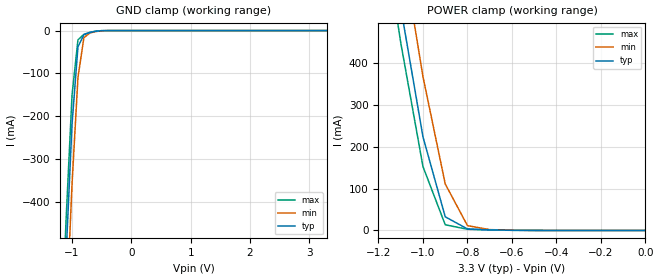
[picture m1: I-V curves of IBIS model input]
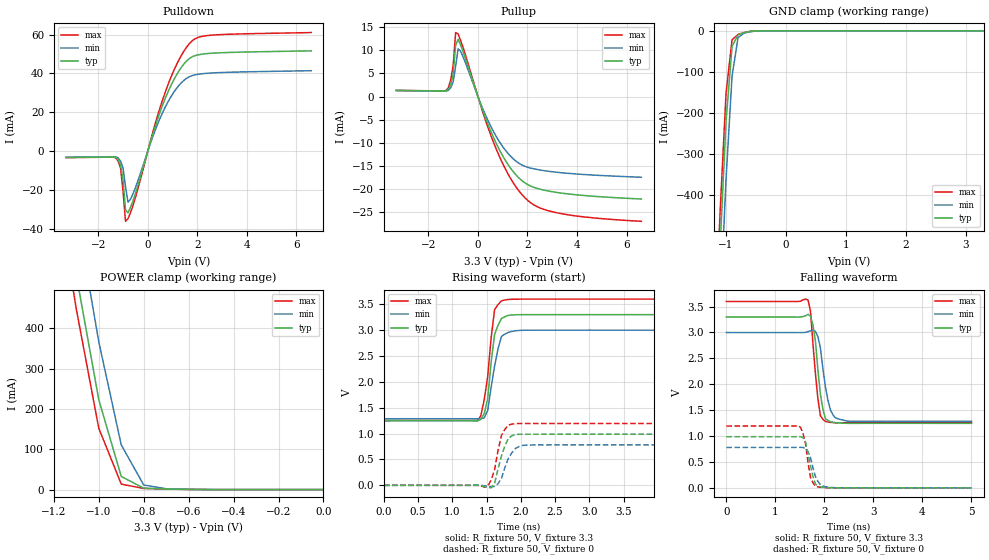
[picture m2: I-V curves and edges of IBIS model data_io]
| TSOP package &  Commercial  Operation
[IBIS Ver]   3.2
[Comment Char]   |_char
[File name]   as7c31026b_tsopc.ibs
[File Rev]   1.0
[Date]   May 19, 2004 3:47:46 PM
[Source]
Alliance Semiconductor Corporation
[Notes]
This model  is for TSOP package &
 Commercial  Operation
[Disclaimer]
Data is for modeling purpose only and is not guaranted.
This IBIS model is provided on an "AS IS" basis and Alliance Semiconductor makes
absolutely no warranty with respect to the information contained
herein.The entire risk as to quality and performance
is with the Customer. ACCORDINGLY, IN NO EVENT SHALL THE COMPANY BE
LIABLE FOR ANY DAMAGES, WHETHER IN CONTRACT OR TORT,INCLUDING ANY
LOST PROFITS OR OTHER INCIDENTAL, CONSEQUENTIAL, EXEMPLARY, OR
PUNITIVE DAMAGES ARISING OUT OF THE USE OR APPLICATION OF THE IBIS
model provided in this package.
[Copyright]
Alliance Semiconductor Corporation
| TSOP Package & Commercial Operation.
[Component]   AS7C31026B_TSOPC
Si_location Pin
Timing_location Pin
[Manufacturer]   Alliance Semiconductor Corporation
[Package]
R_pkg   321.15m   142.5m   499.8m
L_pkg   5.882nH   2.534nH   9.23nH
C_pkg   1.013pF   0.614pF   1.412pF
[Pin] signal_name   model_name
1   A4   input
2   A3   input
3   A2   input
4   A1   input
5   A0   input
6   NCE   input
7   IO0   data_io
8   IO1   data_io
9   IO2   data_io
10   IO3   data_io
11   VCC   POWER
12   GND   GND
13   IO4   data_io
14   IO5   data_io
15   IO6   data_io
16   IO7   data_io
17   NWE   input
18   A15   input
19   A14   input
20   A13   input
21   A12   input
22   NC   NC
23   NC   NC
24   A11   input
25   A10   input
26   A9   input
27   A8   input
28   NC   NC
29   IO8   data_io
30   IO9   data_io
31   IO10   data_io
32   IO11   data_io
33   VCC   POWER
34   GND   GND
35   IO12   data_io
36   IO13   data_io
37   IO14   data_io
38   IO15   data_io
39   NLB   input
40   NUB   input
41   NOE   input
42   A7   input
43   A6   input
44   A5   input
| Models and submodels in the file (2): input (Input), data_io (I/O)
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[Model]   input
Model_type Input
Vinh=2V
Vinl=0.8V
C_comp   4pF   4pF   4pF
[Model Spec]
[Temperature Range] 25   70   0
[Voltage Range]   3.3   3.0   3.6
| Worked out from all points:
|   GND clamp passes 1 mA (typ) near -0.56 V on its own axis
|   POWER clamp passes 1 mA (typ) near -0.65 V on its own axis
[GND Clamp]
-3.3V     -8.605A    -8.678A    -8.569A
-1.2V     -871.8mA   -1.032A    -786.6mA
-1.1V     -525.3mA   -681.9mA   -442.6mA
-1V       -219.6mA   -359.8mA   -151.4mA
-900mV    -38.16mA   -110mA     -21.74mA
-800mV    -9.652mA   -16.68mA   -8.786mA
-700mV    -4.621mA   -5.631mA   -4.129mA
-600mV    -1.581mA   -2.258mA   -1.211mA
-400mV    -22.59uA   -71.08uA   -10.05uA
3.3V      156pA      1.566uA    81.03pA
[POWER Clamp]
-3.3V     8.613A     8.687A     8.576A
-1.2V     879.9mA    1.042A     793.6mA
-1.1V     531.7mA    690.5mA    447.6mA
-1V       222.9mA    366.4mA    152.1mA
-900mV    32.63mA    110.9mA    13.56mA
-800mV    3.618mA    11.48mA    2.851mA
-700mV    1.463mA    2.037mA    1.288mA
0V        156pA      1.542nA    96.3pA
[Model]   data_io
Model_type I/O
Enable Active-High
Polarity Non-Inverting
Vinh=2V
Vinl=0.8V
Vref=1.728V
Vmeas=1.5V
Rref=168
Cref=30pF
C_comp   4pF   4pF   4pF
[Temperature Range] 25   70   0
[Voltage Range]   3.3   3.0   3.6
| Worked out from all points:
|   slope of the pulldown table from 0 to 0.495 V, typ, clamps not added: 24.6 ohm
|   slope of the pullup table from 0 to 0.495 V, typ, clamps not added: 68.8 ohm
|   GND clamp passes 1 mA (typ) near -0.56 V on its own axis
|   POWER clamp passes 1 mA (typ) near -0.65 V on its own axis
|   falling waveform, R_fixture 50, V_fixture 3.3: 20-80 % time 137ps typ, 165ps min, 129ps max; typ from 3.3 V to 1.25 V
|   falling waveform, R_fixture 50, V_fixture 0: 20-80 % time 138ps typ, 152ps min, 120ps max; typ from 0.987 V to 0.001 V
|   rising waveform, R_fixture 50, V_fixture 3.3: 20-80 % time 101ps typ, 134ps min, 119ps max; typ from 1.25 V to 3.3 V
|   rising waveform, R_fixture 50, V_fixture 0: 20-80 % time 131ps typ, 144ps min, 115ps max; typ from 0 V to 0.988 V
[Pullup]
-3.3V     1.309mA    1.298mA    1.319mA
-1.3V     1.177mA    1.139mA    1.277mA
-1.1V     2.464mA    1.876mA    3.58mA
-1V       4.894mA    3.142mA    6.707mA
-900mV    11.13mA    6.531mA    13.83mA
-800mV    12.37mA    10.31mA    13.53mA
-700mV    11.15mA    9.779mA    12.14mA
700mV     -9.696mA   -8.272mA   -10.85mA
1.3V      -15.38mA   -12.82mA   -17.55mA
1.9V      -18.69mA   -15.11mA   -21.92mA
3.2V      -20.76mA   -16.4mA    -25.17mA
6.6V      -22.17mA   -17.47mA   -27mA
[Pulldown]
-3.3V     -3.25mA    -3.145mA   -3.291mA
-1.3V     -3.123mA   -2.838mA   -3.453mA
-1.1V     -7.003mA   -5.036mA   -8.672mA
-1V       -14.54mA   -8.664mA   -20.63mA
-900mV    -30.21mA   -18.24mA   -36.08mA
-800mV    -31.71mA   -26.22mA   -34.76mA
-700mV    -28.96mA   -24.78mA   -31.66mA
700mV     27.02mA    22.56mA    30.19mA
1.2V      40.13mA    32.95mA    45.56mA
1.7V      47.87mA    38.44mA    55.66mA
2.6V      50.42mA    40.25mA    59.72mA
6.6V      51.64mA    41.41mA    61.03mA
[GND Clamp]
-3.3V     -8.605A    -8.678A    -8.569A
-1.2V     -871.8mA   -1.032A    -786.6mA
-1.1V     -525.3mA   -681.9mA   -442.6mA
-1V       -219.6mA   -359.8mA   -151.4mA
-900mV    -38.16mA   -110mA     -21.74mA
-800mV    -9.652mA   -16.68mA   -8.786mA
-700mV    -4.621mA   -5.631mA   -4.129mA
-600mV    -1.581mA   -2.258mA   -1.211mA
-400mV    -22.59uA   -71.08uA   -10.05uA
3.3V      156pA      1.566uA    81.03pA
[POWER Clamp]
-3.3V     8.613A     8.687A     8.576A
-1.2V     879.9mA    1.042A     793.6mA
-1.1V     531.7mA    690.5mA    447.6mA
-1V       222.9mA    366.4mA    152.1mA
-900mV    32.63mA    110.9mA    13.56mA
-800mV    3.618mA    11.48mA    2.851mA
-700mV    1.463mA    2.037mA    1.288mA
0V        156pA      1.542nA    96.3pA
[Falling Waveform]
R_fixture=50
V_fixture=3.3
V_fixture_min=3.0
V_fixture_max=3.6
0s        3.3V       3V         3.6V
1.667ns   3.351V     3.017V     3.628V
1.717ns   3.312V     3.032V     3.402V
1.768ns   3.14V      3.048V     2.771V
1.869ns   2.263V     2.916V     1.713V
1.919ns   1.806V     2.699V     1.39V
2.02ns    1.339V     1.954V     1.283V
2.121ns   1.279V     1.51V      1.265V
2.323ns   1.253V     1.32V      1.256V
5ns       1.247V     1.288V     1.255V
[Falling Waveform]
R_fixture=50
V_fixture=0
V_fixture_min=0
V_fixture_max=0
0s        987.1mV    780.3mV    1.194V
1.465ns   991.4mV    782.8mV    1.199V
1.515ns   988.3mV    783.2mV    1.167V
1.616ns   884.2mV    759.7mV    851mV
1.667ns   650.4mV    697.8mV    480.1mV
1.717ns   425.3mV    587.2mV    200.8mV
1.818ns   72.24mV    218mV      30.49mV
1.919ns   18.85mV    61.55mV    11.86mV
2.172ns   3.007mV    6.68mV     1.845mV
5ns       1.203mV    1.221mV    1.233mV
[Rising Waveform]
R_fixture=50
V_fixture=3.3
V_fixture_min=3.0
V_fixture_max=3.6
0s        1.246V     1.287V     1.254V
1.364ns   1.244V     1.286V     1.253V
1.414ns   1.273V     1.289V     1.339V
1.465ns   1.383V     1.303V     1.653V
1.515ns   1.672V     1.446V     2.098V
1.566ns   2.377V     1.893V     2.85V
1.616ns   2.915V     2.304V     3.393V
1.717ns   3.224V     2.878V     3.564V
2.02ns    3.298V     2.996V     3.598V
5ns       3.298V     2.998V     3.598V
[Rising Waveform]
R_fixture=50
V_fixture=0
V_fixture_min=0
V_fixture_max=0
0s        0V         0V         0V
1.515ns   -39.5mV    -15.58mV   -16.28mV
1.566ns   -47.94mV   -27.89mV   101.8mV
1.616ns   36.55mV    -19.97mV   302mV
1.717ns   571.3mV    136.7mV    965.1mV
1.818ns   909.9mV    523.2mV    1.166V
1.869ns   956.2mV    630.6mV    1.183V
1.97ns    986.7mV    748.6mV    1.194V
2.121ns   987.9mV    779mV      1.194V
5ns       988.3mV    781.6mV    1.195V
[Ramp]
R_load=50
dV/dt_r   5.930E-1/1.286E-10   4.690E-1/1.443E-10   7.167E-1/1.055E-10
dV/dt_f   1.232E+0/1.330E-10   1.027E+0/1.597E-10   1.407E+0/1.286E-10
|[End   data_io
